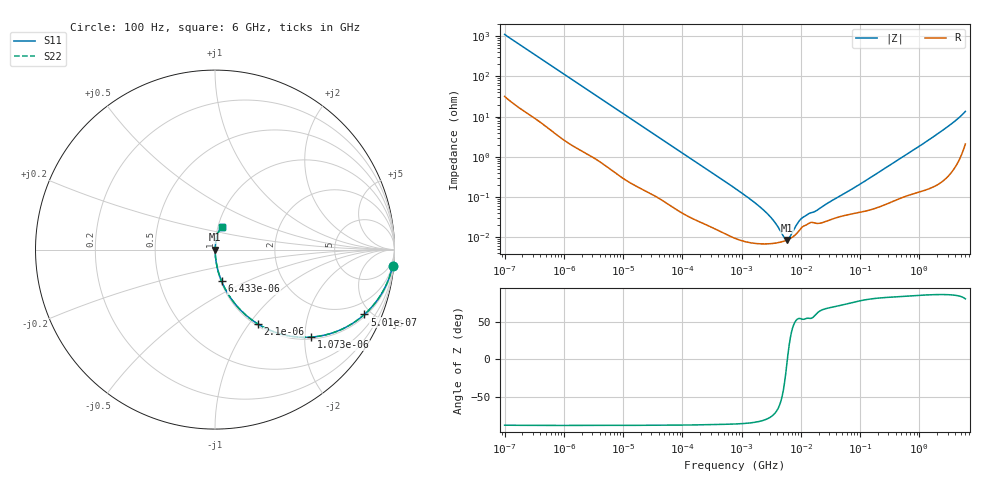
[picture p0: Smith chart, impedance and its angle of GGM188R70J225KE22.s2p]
!Murata Part Number: GGM188R70J225KE22
!These Parameters are Measured in Series Mode Connection
!Data Generated on Jun 19, 2026
!  o--ll--o
!Port1  Port2
!  o------o
!Operation Temp=25[degC], DC Bias Voltage=0[V]
!Freq. Start=100[Hz] Stop=6[GHz] 401[Steps]
# Hz S RI R 50
!Freq.(Hz) S11(Real) S11(Imag) S21(Real) S21(Imag) S12(Real) S12(Imag) S22(Real) S22(Imag)
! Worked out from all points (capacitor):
!   401 points, 100 Hz to 6 GHz, reference 50 ohm
!   read as one part in series: C = 1.42 uF near 109 Hz
!   lowest |Z| = 8.46 mohm at 5.809 MHz (marker M1)
!   series resonance near 5.931 MHz, so ESL is about 510 pH
!   S11 on the Smith chart (normalised r, x): 100 Hz: 2, -22; 501 Hz: 1.11, -4.55; 1.073 kHz: 1.05, -2.15; 2.1 kHz: 1.03, -1.11; 6.433 kHz: 1.01, -0.37; 6 GHz: 1.04, +0.27
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100  0.9895 -0.0886  0.0105 0.0886  0.0105 0.0886  0.9895 -0.0886
268  0.9416 -0.2219  0.0584 0.2219  0.0584 0.2219  0.9416 -0.2219
501  0.8322 -0.3615  0.1678 0.3615  0.1678 0.3615  0.8322 -0.3615
717  0.7145 -0.4401  0.2855 0.4401  0.2855 0.4401  0.7145 -0.4401
1073  0.535 -0.4876  0.465 0.4876  0.465 0.4876  0.535 -0.4876
2008  0.2558 -0.4245  0.7442 0.4245  0.7442 0.4245  0.2558 -0.4245
2100  0.2399 -0.415  0.7601 0.415  0.7601 0.415  0.2399 -0.415
3437  0.1104 -0.3008  0.8896 0.3008  0.8896 0.3008  0.1104 -0.3008
6433  0.037 -0.1766  0.963 0.1766  0.963 0.1766  0.037 -0.1766
14402  0.0089 -0.0823  0.9911 0.0823  0.9911 0.0823  0.0089 -0.0823
40335  0.00183 -0.0302  0.9982 0.0302  0.9982 0.0302  0.00183 -0.0302
774597  9.56e-05 -0.00164  0.9999 0.00164  0.9999 0.00164  9.56e-05 -0.00164
2481164  6.77e-05 -0.000433  0.9999 0.000433  0.9999 0.000433  6.77e-05 -0.000433
3549919  7e-05 -0.000236  0.9999 0.000236  0.9999 0.000236  7e-05 -0.000236
5079039  7.83e-05 -6.86e-05  0.9999 6.86e-05  0.9999 6.86e-05  7.83e-05 -6.86e-05
5809218  8.41e-05 -9.1e-06  0.9999 9.1e-06  0.9999 9.1e-06  8.41e-05 -9.1e-06
6644369  9.25e-05 5.05e-05  0.9999 -5.05e-05  0.9999 -5.05e-05  9.25e-05 5.05e-05
9941735  0.000161 0.000227  0.9998 -0.000227  0.9998 -0.000227  0.000161 0.000227
1.555665e7  0.000233 0.000338  0.9998 -0.000338  0.9998 -0.000338  0.000233 0.000338
3.124326e8  0.000747 0.00602  0.9993 -0.00602  0.9993 -0.00602  0.000747 0.00602
2.142435e9  0.00363 0.039  0.9964 -0.039  0.9964 -0.039  0.00363 0.039
6e9  0.037 0.1262  0.963 -0.1262  0.963 -0.1262  0.037 0.1262
